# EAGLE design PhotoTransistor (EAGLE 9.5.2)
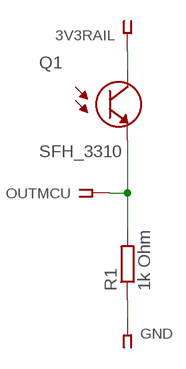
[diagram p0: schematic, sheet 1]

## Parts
3V3RAIL  SSW-101-02-G-S  [SSW-101-02-G-S]
GND  SSW-101-02-G-S  [SSW-101-02-G-S]
OUTMCU  SSW-101-02-G-S  [SSW-101-02-G-S]
Q1  SFH_3310  [XDCR_SFH_3310]
R1  1k Ohm  R-EU_M1206  [M1206]

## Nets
N$1: 3V3RAIL.1 Q1.2(C)
N$2: GND.1 R1.1
N$3: OUTMCU.1 Q1.1(E) R1.2

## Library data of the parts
3V3RAIL GND OUTMCU = con-samtec:SSW-101-02-G-S: THROUGH-HOLE .025" SQ POST SOCKET; MF: Samtec Inc.; MPN: SSW-101-02-G-S; OC_FARNELL: unknown; OC_NEWARK: 11P9336
Q1 = SFH_3310:SFH_3310: Ambient Light Sensor Phototransistor Chip Silicon 570nm 2-Pin T-1; AVAILABILITY: Unavailable; DESCRIPTION: Phototransistor 570nm Top View Radial; MF: OSRAM Opto; MP: SFH 3310; PACKAGE: Radial Osram Opto; PRICE: None
R1 = rcl:R-EU_: RESISTOR, European symbol; SPICEPREFIX: R

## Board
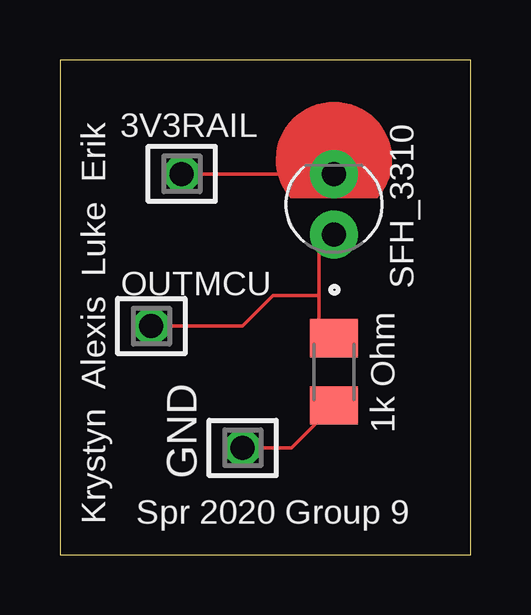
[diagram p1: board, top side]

Size 17.12 x 20.62 mm. Coordinates in mm from the lower left corner, seen from the top.
Outline: 0,0 17.12,0 17.12,20.62 0,20.62 0,0
Copper layers (1*16): Top 0.035mm / dielectric 1.5mm / Bottom 0.035mm
Design rules "default": minimum track width 6mil, minimum drill 0.35mm, track to track 6mil, track to pad 6mil, pad to pad 6mil, via to via 6mil, smd to smd 6mil, copper to edge 40mil, drill to drill 6mil, minimum pad ring 10mil, minimum via ring 8mil, stop-mask expansion 4mil, vias tented up to drill 0mil, thermal gap 10mil

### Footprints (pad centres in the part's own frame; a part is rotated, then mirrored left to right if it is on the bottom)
SSW-101-02-G-S = drill 1 pad 1.5 octagon: 1 0,0
XDCR_SFH_3310 = drill 1 pad 2: 1 -1.27,0; 2 1.27,0
M1206 = smd 1.6 x 2: 1 -1.4,0; 2 1.4,0

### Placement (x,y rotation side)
3V3RAIL  5.08,15.88 0 top
GND  7.62,4.45 0 top
OUTMCU  3.81,9.53 0 top
Q1  11.43,14.61 90 top
R1  11.43,7.62 90 top

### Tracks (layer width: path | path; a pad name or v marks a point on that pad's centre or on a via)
N$1
  Top 0.152: 3V3RAIL.1 Q1.2
N$2
  Top 0.152: R1.1 9.65,4.45 GND.1
N$3
  Top 0.152: Q1.1 10.79,12.7 10.79,10.8 | 10.79,10.8 10.79,9.65 R1.2 | OUTMCU.1 7.62,9.53 8.89,10.8 10.79,10.8

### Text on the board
tNames: Krystyn Alexis Luke Erik | Spr 2020 Group 9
